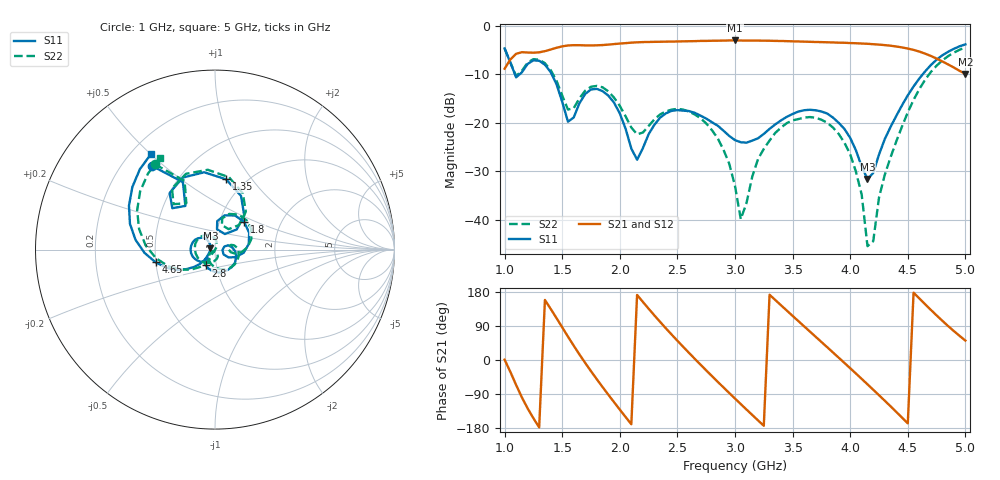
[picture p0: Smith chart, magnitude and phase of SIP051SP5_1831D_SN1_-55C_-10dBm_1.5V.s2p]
# GHz  S  dB  R  50
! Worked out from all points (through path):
!   81 points, 1 GHz to 5 GHz, reference 50 ohm
!   highest |S21| = -3.05 dB at 3 GHz (marker M1); lowest = -9.9 dB at 5 GHz (marker M2)
!   lowest |S11| = -31.6 dB at 4.15 GHz (marker M3), VSWR 1.05, Z = 47.5 + j0.638 ohm
!   |S11| at or under -10 dB: 1.09 GHz to 1.131 GHz (41.16 MHz wide, 3.71 % of centre); 1.409 GHz to 4.63 GHz (3.222 GHz wide, 107 % of centre)
!   |S22| runs from -45.4 to -4.5 dB; largest |S21 - S12| = 0.0019
!   S11 on the Smith chart (normalised r, x): 1 GHz: 0.32, +0.46; 1.35 GHz: 0.82, +0.76; 1.8 GHz: 1.31, +0.42; 2.8 GHz: 0.89, -0.16; 4.65 GHz: 0.50, -0.08; 5 GHz: 0.28, +0.50
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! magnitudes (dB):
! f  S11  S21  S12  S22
! 1 GHz  -4.7  -8.9  -8.9  -4.7
! 1.1 GHz  -10.6  -5.8  -5.8  -10.4
! 1.35 GHz  -8.0  -5.3  -5.2  -7.7
! 1.55 GHz  -19.8  -4.1  -4.1  -17.3
! 1.7 GHz  -14.1  -4.1  -4.1  -13.4
! 1.8 GHz  -13.0  -4.0  -4.0  -12.4
! 1.95 GHz  -15.8  -3.8  -3.8  -14.8
! 2.15 GHz  -27.6  -3.4  -3.4  -22.4
! 2.35 GHz  -18.9  -3.3  -3.3  -18.3
! 2.8 GHz  -19.9  -3.1  -3.1  -21.5
! 3 GHz  -23.6  -3.0  -3.1  -33.0
! 3.05 GHz  -24.0  -3.1  -3.0  -39.8
! 3.3 GHz  -21.2  -3.1  -3.1  -23.6
! 3.7 GHz  -17.4  -3.4  -3.4  -19.0
! 4 GHz  -23.1  -3.6  -3.6  -26.5
! 4.1 GHz  -29.0  -3.7  -3.7  -34.8
! 4.15 GHz  -31.6  -3.7  -3.7  -45.4
! 4.2 GHz  -30.3  -3.8  -3.8  -44.4
! 4.25 GHz  -26.5  -3.9  -3.9  -35.4
! 4.35 GHz  -20.9  -4.1  -4.1  -27.1
! 4.65 GHz  -9.4  -5.8  -5.8  -11.2
! 5 GHz  -3.9  -9.9  -9.9  -4.5
